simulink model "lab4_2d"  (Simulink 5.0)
settings: Solver=FixedStepDiscrete  StartTime=0.0  StopTime=2*1e-3  FixedStep=T  RelTol=1e-3
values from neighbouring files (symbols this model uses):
  T = 1/Fsamp    (= 0.0001)    [lab4_4.m]

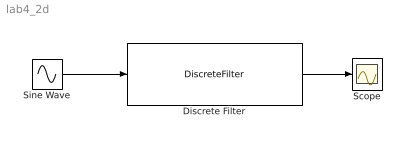
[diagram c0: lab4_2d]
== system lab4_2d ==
  Discrete Filter : DiscreteFilter  Numerator="[2  1]"  Denominator="[1  -1.8*cos(pi/16)  0.81]"  SampleTime=T
  Scope : Scope
  Sine Wave : Sin  Frequency=2*pi*1.6e3  Phase=pi/3  SampleTime=T
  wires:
  Discrete Filter/1 -> Scope/1
  Sine Wave/1 -> Discrete Filter/1
